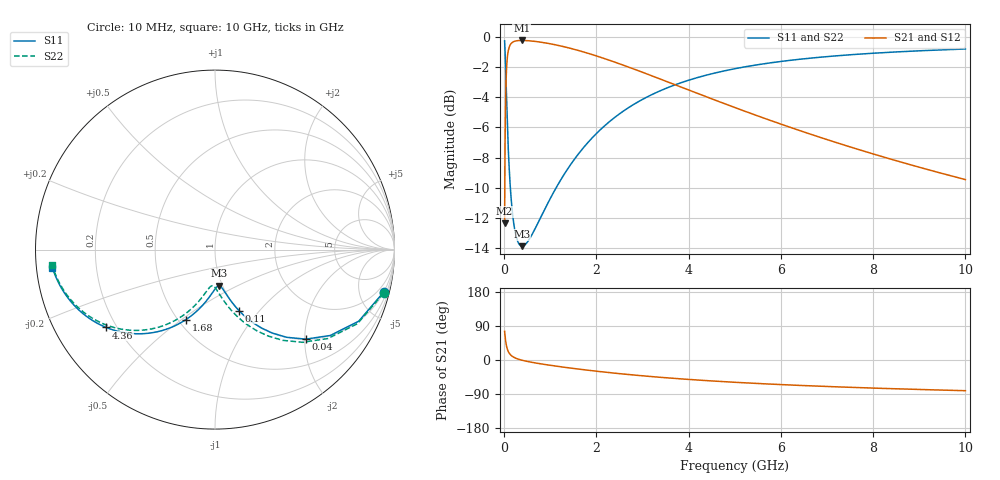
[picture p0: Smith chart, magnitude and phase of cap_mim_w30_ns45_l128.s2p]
! Created Wed Nov  4 11:45:59 2020
# ghz S ma R 50
! 2 Port Network Data from SP1.SP block
! freq  magS11  angS11  magS21  angS21  magS12  angS12  magS22  angS22
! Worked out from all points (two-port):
!   1000 points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, 10 MHz to 10 GHz, reference 50 ohm
!   highest |S21| = -0.24 dB at 380 MHz (marker M1); lowest = -12.4 dB at 10 MHz (marker M2)
!   |S21| within 3 dB of the highest: 39.07 MHz to 3.761 GHz (3.722 GHz wide, 196 % of centre)
!   lowest |S11| = -13.9 dB at 390 MHz (marker M3), VSWR 1.51, Z = 48 - j20.2 ohm
!   |S11| at or under -10 dB: 134.7 MHz to 1.126 GHz (991.3 MHz wide, 157 % of centre)
!   |S22| runs from -13.9 to -0.3 dB; largest |S21 - S12| = 0
!   S11 on the Smith chart (normalised r, x): 10 MHz: 1.01, -8.01; 40 MHz: 1.00, -2.02; 110 MHz: 1.00, -0.79; 1.68 GHz: 0.55, -0.52; 4.36 GHz: 0.16, -0.31; 10 GHz: 0.05, -0.06
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0.01  0.9701 -14.0  0.2411 75.6  0.2411 75.6  0.9701 -14.5
0.04  0.7104 -44.6  0.6992 44.0  0.6992 44.0  0.7102 -46.7
0.07  0.5079 -59.3  0.8559 28.3  0.8559 28.3  0.5076 -62.8
0.09  0.4241 -64.8  0.8999 22.2  0.8999 22.2  0.4236 -69.2
0.11  0.3658 -68.5  0.9248 17.9  0.9248 17.9  0.3652 -73.8
0.13  0.3241 -71.2  0.9401 14.8  0.9401 14.8  0.3234 -77.2
0.16  0.2812 -74.0  0.9536 11.2  0.9536 11.2  0.2804 -81.1
0.22  0.2343 -77.7  0.966 6.5  0.966 6.5  0.2334 -86.3
0.29  0.211 -80.6  0.9713 2.9  0.9713 2.9  0.2099 -90.2
0.38  0.2028 -83.7  0.9729 -0.4  0.9729 -0.4  0.2016 -93.7
0.39  0.2027 -84.0  0.9729 -0.7  0.9729 -0.7  0.2016 -94.0
0.56  0.2155 -89.0  0.9698 -5.2  0.9698 -5.2  0.2145 -98.4
0.93  0.2781 -98.2  0.9528 -12.7  0.9528 -12.7  0.2773 -105.3
1.3  0.3504 -105.8  0.9273 -19.1  0.9273 -19.1  0.3497 -111.3
1.68  0.4224 -112.6  0.895 -25.0  0.895 -25.0  0.4219 -117.0
2.45  0.5487 -124.1  0.8195 -35.4  0.8195 -35.4  0.5483 -127.2
3.34  0.6584 -134.7  0.7293 -45.2  0.7293 -45.2  0.6581 -137.0
4.36  0.7452 -144.4  0.6351 -54.2  0.6351 -54.2  0.7449 -146.2
5.01  0.7847 -149.4  0.5827 -58.9  0.5827 -58.9  0.7845 -151.0
6.67  0.8511 -159.7  0.4745 -68.3  0.4745 -68.3  0.8509 -160.8
8.34  0.8887 -167.5  0.3953 -75.4  0.3953 -75.4  0.8886 -168.4
10  0.9114 -173.7  0.3368 -81.0  0.3368 -81.0  0.9113 -174.4
